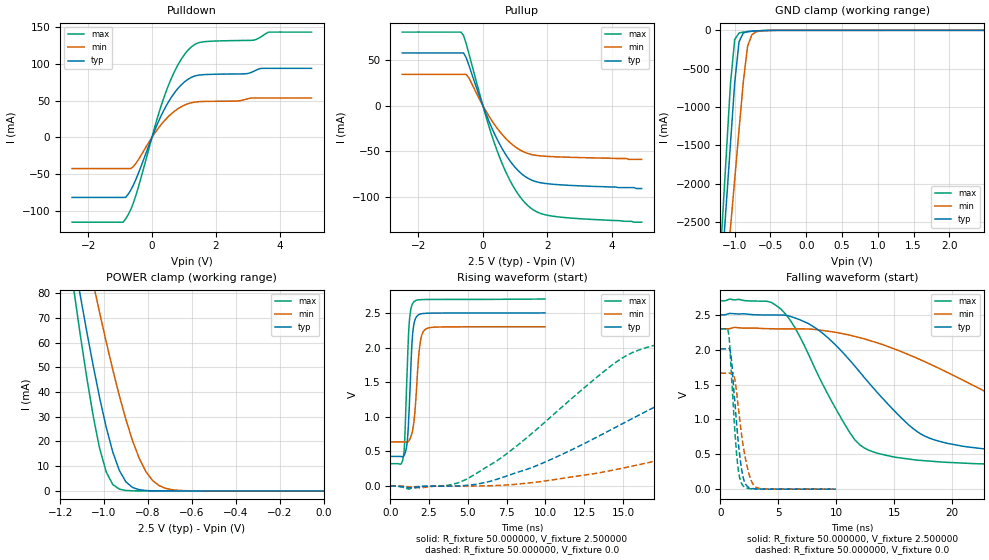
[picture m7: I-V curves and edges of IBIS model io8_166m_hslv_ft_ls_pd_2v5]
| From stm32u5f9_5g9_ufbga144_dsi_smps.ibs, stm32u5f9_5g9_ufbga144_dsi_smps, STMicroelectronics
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|   Model io8_166m_hslv_ft_ls_pd_2v5
[Model]  io8_166m_hslv_ft_ls_pd_2v5
Model_type I/O
Polarity   Non-Inverting
Enable   Active-Low
Vinl =   0.750000V
Vinh =   1.750000V
Vmeas =  1.250000V
Cref =   50.000000pF
Rref =   100.000000M
Vref =   0.0V
C_comp   3.458600pF   3.457900pF   3.495500pF
[Temperature Range]   25.000000   0.140000k   -40.000000
[Pullup Reference]   2.500000V   2.300000V   2.700000V
[Pulldown Reference]   0.0V   0.0V   0.0V
[POWER Clamp Reference]   2.500000V   2.300000V   2.700000V
[GND Clamp Reference]   0.0V   0.0V   0.0V
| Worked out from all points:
|   slope of the pulldown table from 0 to 0.375 V, typ, clamps not added: 10.1 ohm
|   slope of the pullup table from 0 to 0.375 V, typ, clamps not added: 11.7 ohm
|   GND clamp passes 1 mA (typ) near -0.50 V on its own axis
|   POWER clamp passes 1 mA (typ) near -0.86 V on its own axis
|   rising waveform, R_fixture 50.000000, V_fixture 2.500000: 20-80 % time 247ps typ, 327ps min, 231ps max; typ from 0.427 V to 2.5 V
|   rising waveform, R_fixture 50.000000, V_fixture 0.0: 20-80 % time 11.1ns typ, 20ns min, 7.42ns max; typ from 0 V to 2.01 V
|   falling waveform, R_fixture 50.000000, V_fixture 2.500000: 20-80 % time 7.02ns typ, 13.9ns min, 4.49ns max; typ from 2.5 V to 0.427 V
|   falling waveform, R_fixture 50.000000, V_fixture 0.0: 20-80 % time 657ps typ, 860ps min, 541ps max; typ from 2.01 V to 0 V
[Pulldown]
|Voltage   I(typ)   I(min)   I(max)
-2.5V     -81.61mA   -42.31mA   -115.3mA
-900mV    -81.61mA   -42.31mA   -115.3mA
-820mV    -81.43mA   -42.31mA   -110.6mA
-500mV    -56.95mA   -35.08mA   -78.57mA
140mV     15.18mA    9.02mA     22.02mA
460mV     44mA       25.98mA    64.38mA
860mV     68.91mA    40.27mA    102.2mA
1.26V     82.21mA    47.42mA    124mA
1.66V     85.54mA    48.99mA    130.3mA
3.18V     89.84mA    53.64mA    132.3mA
3.66V     94.01mA    53.64mA    143.3mA
5V        94.01mA    53.64mA    143.3mA
[Pullup]
|Voltage   I(typ)   I(min)   I(max)
-2.5V     57.98mA    34.47mA    80.92mA
-680mV    57.98mA    34.47mA    80.92mA
-600mV    57.98mA    34.47mA    77.15mA
-440mV    45.11mA    30.85mA    58.07mA
120mV     -11.17mA   -7.509mA   -14.95mA
520mV     -42.32mA   -28.36mA   -56.93mA
760mV     -56.64mA   -37.85mA   -76.55mA
1V        -67.83mA   -45.13mA   -92.22mA
1.48V     -81.29mA   -53.4mA    -112.4mA
1.8V      -84.73mA   -55.19mA   -118.5mA
2.28V     -86.63mA   -56.16mA   -121.9mA
4.92V     -91mA      -59mA      -128mA
[GND_clamp]
|Voltage   I(typ)   I(min)   I(max)
-2.5V     -9.641A    -9.693A    -9.352A
-1.18V    -3.114A    -3.874A    -2.614A
-1.12V    -2.301A    -3.23A     -1.656A
-1.06V    -1.489A    -2.587A    -706.2mA
-1V       -685.8mA   -1.945A    -119.3mA
-940mV    -149.8mA   -1.304A    -34.74mA
-880mV    -35.55mA   -672.6mA   -23.08mA
-820mV    -16.21mA   -206.4mA   -17.29mA
-760mV    -10.59mA   -57.56mA   -12.42mA
-700mV    -7.163mA   -18.75mA   -8.254mA
-400mV    -112.4uA   -385.2uA   -53.47uA
2.48V     63.1uA     48.03uA    77.39uA
[POWER_clamp]
|Voltage   I(typ)   I(min)   I(max)
-2.49V    881mA      773.1mA    1.07A
-1.14V    95.25mA    122.7mA    82.82mA
-1.11V    79.9mA     109.7mA    64.14mA
-1.05V    50.87mA    84.26mA    30.57mA
-1.02V    37.63mA    72.04mA    17.17mA
-990mV    25.71mA    60.25mA    7.621mA
-930mV    8.217mA    38.43mA    713.9uA
-900mV    3.624mA    28.77mA    182.8uA
-840mV    490.7uA    13.24mA    11.35uA
-780mV    56.55uA    4.324mA    699nA
-660mV    716.7nA    226uA      9.784nA
0V        0A         19.53nA    0A
[Ramp]
| variable   typ   min   max
dV/dt_r  1.20630/11.05557n   0.99744/19.93746n   1.37748/7.40458n
dV/dt_f  1.24322/7.01223n   0.99725/13.87150n   1.42604/4.48141n
R_load = 50.000000
[Rising Waveform]
R_fixture= 50.000000
V_fixture= 2.500000
V_fixture_min= 2.300000
V_fixture_max= 2.700000
|time   V(typ)   V(min)   V(max)
0s        427.5mV    637.3mV    322.6mV
840.8ps   428.2mV    637.3mV    415.8mV
940.9ps   468.5mV    636.8mV    715.7mV
1.101ns   655.6mV    634.9mV    1.737V
1.201ns   1.031V     652mV      2.287V
1.381ns   1.994V     750.3mV    2.6V
1.522ns   2.334V     922.6mV    2.66V
1.902ns   2.481V     2.025V     2.69V
2.262ns   2.494V     2.262V     2.693V
9.97ns    2.499V     2.299V     2.699V
[Rising Waveform]
R_fixture= 50.000000
V_fixture= 0.0
V_fixture_min= 0.0
V_fixture_max= 0.0
|time   V(typ)   V(min)   V(max)
0s        2.072nV    118.4nV    2.101nV
3.604ns   -1.316mV   -1.021mV   7.171mV
5.205ns   15.24mV    161uV      135.3mV
9.61ns    310.6mV    61.82mV    851.9mV
15.62ns   976mV      289.1mV    1.928V
21.22ns   1.578V     579.2mV    2.177V
25.63ns   1.799V     818.6mV    2.239V
38.04ns   1.961V     1.376V     2.288V
54.05ns   2.002V     1.578V     2.295V
199.4ns   2.01V      1.663V     2.296V
[Falling Waveform]
R_fixture= 50.000000
V_fixture= 2.500000
V_fixture_min= 2.300000
V_fixture_max= 2.700000
|time   V(typ)   V(min)   V(max)
0s        2.499V     2.299V     2.699V
5.205ns   2.496V     2.298V     2.585V
6.406ns   2.456V     2.297V     2.324V
8.408ns   2.289V     2.284V     1.646V
12.01ns   1.684V     2.172V     639mV
16.42ns   899.1mV    1.917V     428.4mV
19.22ns   672.8mV    1.705V     387.4mV
29.23ns   501.3mV    982.1mV    339mV
45.25ns   445.7mV    741.7mV    325.3mV
199.4ns   427.5mV    637.3mV    322.6mV
[Falling Waveform]
R_fixture= 50.000000
V_fixture= 0.0
V_fixture_min= 0.0
V_fixture_max= 0.0
|time   V(typ)   V(min)   V(max)
0s        2.01V      1.663V     2.296V
620.6ps   2.01V      1.663V     2.296V
780.8ps   2.013V     1.663V     2.122V
880.9ps   1.945V     1.662V     1.847V
1.181ns   1.373V     1.625V     1.008V
1.461ns   818.6mV    1.296V     396.1mV
1.922ns   201.3mV    671.4mV    56.61mV
2.482ns   22.06mV    211.5mV    7.437mV
3.083ns   3.155mV    27.14mV    1.965mV
9.97ns    2.072nV    118.4nV    2.101nV
